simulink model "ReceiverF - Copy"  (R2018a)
settings: Solver=FixedStepDiscrete  StartTime=0.0  StopTime=2  RelTol=1e-3
undefined symbols (not defined in the file): DiscIntNeverNeededParam
libraries: simulink x54, dspsigops x27, commutil2 x6, c280xlib x2, c2803xlib x1, dspstat3 x1

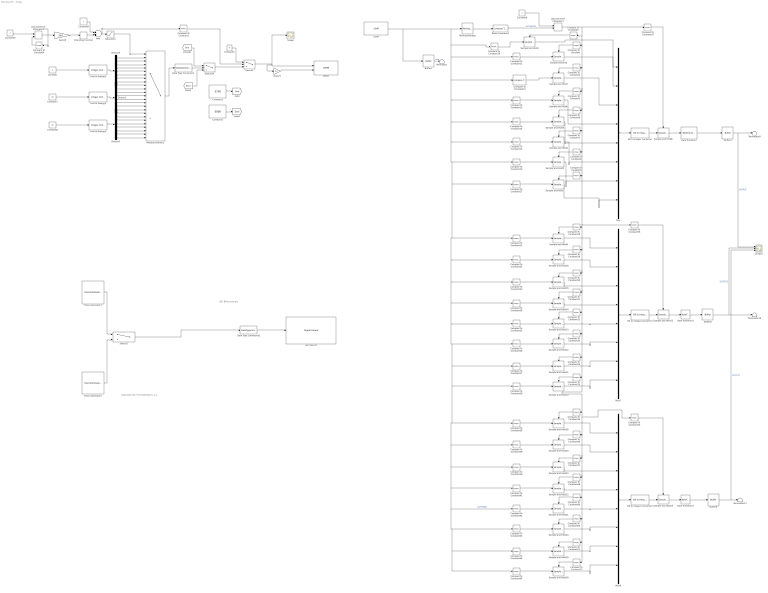
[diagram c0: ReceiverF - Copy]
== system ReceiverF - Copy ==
  note: Copyright 2017 The MathWorks, Inc.
  note: LED Blink example
  Add : Sum
  Bit to Integer Converter : commutil2/Bit to Integer Converter  nbits=8  bitOrder=MSB first  signedOutputValues=Unsigned  outDtype=Inherit via internal rule  outDtypeSigned=Inherit via internal rule
  Bit to Integer Converter4 : commutil2/Bit to Integer Converter  nbits=8  bitOrder=MSB first  signedOutputValues=Unsigned  outDtype=Inherit via internal rule  outDtypeSigned=Inherit via internal rule
  Bit to Integer Converter5 : commutil2/Bit to Integer Converter  nbits=8  bitOrder=MSB first  signedOutputValues=Unsigned  outDtype=Inherit via internal rule  outDtypeSigned=Inherit via internal rule
  Buffer1 : Buffer  N=500  OutputFrames=off
  Buffer4 : Buffer  N=5  OutputFrames=off
  Buffer8 : Buffer  N=5  OutputFrames=off
  Buffer9 : Buffer  N=5  OutputFrames=off
  Compare To Constant : simulink/Logic and Bit Operations/Compare To Constant  relop=>=  const=1  OutDataTypeStr=boolean
  Compare To Constant1 : simulink/Logic and Bit Operations/Compare To Constant  relop=>=  const=25  OutDataTypeStr=boolean
  Compare To Constant10 : simulink/Logic and Bit Operations/Compare To Constant  relop=>=  const=24  OutDataTypeStr=boolean
  Compare To Constant{11..18,21..28,38..45} (24 alike) : simulink/Logic and Bit Operations/Compare To Constant  relop=<=  const=4800  OutDataTypeStr=boolean
  Compare To Constant19 : simulink/Logic and Bit Operations/Compare To Constant  relop=>=  const=8  OutDataTypeStr=boolean
  Compare To Constant2 : simulink/Logic and Bit Operations/Compare To Constant  relop=>=  const=2  OutDataTypeStr=boolean
  Compare To Constant20 : simulink/Logic and Bit Operations/Compare To Constant  relop=>=  const=15  OutDataTypeStr=boolean
  Compare To Constant29 : simulink/Logic and Bit Operations/Compare To Constant  relop=>=  const=9  OutDataTypeStr=boolean
  Compare To Constant3 : simulink/Logic and Bit Operations/Compare To Constant  relop=>=  const=3  OutDataTypeStr=boolean
  Compare To Constant30 : simulink/Logic and Bit Operations/Compare To Constant  relop=>=  const=10  OutDataTypeStr=boolean
  Compare To Constant31 : simulink/Logic and Bit Operations/Compare To Constant  relop=>=  const=11  OutDataTypeStr=boolean
  Compare To Constant32 : simulink/Logic and Bit Operations/Compare To Constant  relop=>=  const=12  OutDataTypeStr=boolean
  Compare To Constant33 : simulink/Logic and Bit Operations/Compare To Constant  relop=>=  const=13  OutDataTypeStr=boolean
  Compare To Constant34 : simulink/Logic and Bit Operations/Compare To Constant  relop=>=  const=14  OutDataTypeStr=boolean
  Compare To Constant35 : simulink/Logic and Bit Operations/Compare To Constant  relop=>=  const=24  OutDataTypeStr=boolean
  Compare To Constant36 : simulink/Logic and Bit Operations/Compare To Constant  relop=>=  const=16  OutDataTypeStr=boolean
  Compare To Constant37 : simulink/Logic and Bit Operations/Compare To Constant  relop=>=  const=23  OutDataTypeStr=boolean
  Compare To Constant4 : simulink/Logic and Bit Operations/Compare To Constant  relop=>  const=1  OutDataTypeStr=uint8
  Compare To Constant46 : simulink/Logic and Bit Operations/Compare To Constant  relop=>=  const=17  OutDataTypeStr=boolean
  Compare To Constant47 : simulink/Logic and Bit Operations/Compare To Constant  relop=>=  const=18  OutDataTypeStr=boolean
  Compare To Constant48 : simulink/Logic and Bit Operations/Compare To Constant  relop=>=  const=19  OutDataTypeStr=boolean
  Compare To Constant49 : simulink/Logic and Bit Operations/Compare To Constant  relop=>=  const=20  OutDataTypeStr=boolean
  Compare To Constant5 : simulink/Logic and Bit Operations/Compare To Constant  relop=>  const=0  OutDataTypeStr=boolean
  Compare To Constant50 : simulink/Logic and Bit Operations/Compare To Constant  relop=>=  const=21  OutDataTypeStr=boolean
  Compare To Constant51 : simulink/Logic and Bit Operations/Compare To Constant  relop=>=  const=22  OutDataTypeStr=boolean
  Compare To Constant52 : simulink/Logic and Bit Operations/Compare To Constant  relop=>=  const=24  OutDataTypeStr=boolean
  Compare To Constant6 : simulink/Logic and Bit Operations/Compare To Constant  relop=>=  const=4  OutDataTypeStr=boolean
  Compare To Constant7 : simulink/Logic and Bit Operations/Compare To Constant  relop=>=  const=5  OutDataTypeStr=boolean
  Compare To Constant8 : simulink/Logic and Bit Operations/Compare To Constant  relop=>=  const=6  OutDataTypeStr=boolean
  Compare To Constant9 : simulink/Logic and Bit Operations/Compare To Constant  relop=>=  const=7  OutDataTypeStr=boolean
  Constant : Constant  Value=6
  Constant1 : Constant  Value=3750  VectorParams1D=off
  Constant2 : Constant  Value=5000  VectorParams1D=off
  Constant4 : Constant
  Constant5 : Constant  Value=0  VectorParams1D=off  SampleTime=-1
  Constant6 : Constant  OutDataTypeStr=int8  SampleTime=-1
  Constant7 : Constant  Value=20  OutDataTypeStr=int8  SampleTime=100e-6
  Constant8 : Constant  Value=33  OutDataTypeStr=int8  SampleTime=100e-6
  Constant9 : Constant  SampleTime=100e-6
  Cost of Energy1 : commutil2/Integer to Bit Converter  nbits=8  signedInputValues=Unsigned  bitOrder=MSB first  outDtype=Inherit via internal rule
  Cost of Energy2 : commutil2/Integer to Bit Converter  nbits=8  signedInputValues=Unsigned  bitOrder=MSB first  outDtype=Inherit via internal rule
  Cost of Energy3 : commutil2/Integer to Bit Converter  nbits=8  signedInputValues=Unsigned  bitOrder=MSB first  outDtype=Inherit via internal rule
  Data Type Conversion : DataTypeConversion  OutDataTypeStr=boolean
  Data Type Conversion1 : DataTypeConversion  Commented=on  OutDataTypeStr=boolean
  Demux1 : Demux  Outputs=8
  Demux2 : Demux  Outputs=8
  Demux3 : Demux  Outputs=8
  Discrete-Time Integrator1 : DiscreteIntegrator  gainval=1e3  ExternalReset=falling  SampleTime=400e-6  ICPrevOutput=DiscIntNeverNeededParam  ICPrevScaledInput=DiscIntNeverNeededParam
  Discrete-Time Integrator2 : DiscreteIntegrator  gainval=1  ExternalReset=rising  SampleTime=100e-6  ShowStatePort=on  ICPrevOutput=DiscIntNeverNeededParam  ICPrevScaledInput=DiscIntNeverNeededParam
  Gain26 : Gain  Gain=1e3
  Gain27 : Gain  Gain=0.5
  LED RIGHT1 : c2803xlib/Digital Output  Commented=on  GPIO_Number=GPIO32~GPIO39  GPIO_Bit0=off  GPIO_BIT0_Toggle=off  GPIO_Bit1=off  GPIO_BIT1_Toggle=off  GPIO_Bit2=on  GPIO_BIT2_Toggle=off  GPIO_Bit3=off  GPIO_BIT3_Toggle=off  GPIO_Bit4=off  GPIO_BIT4_Toggle=off  GPIO_Bit5=off  GPIO_BIT5_Toggle=off  GPIO_Bit6=off  GPIO_BIT6_Toggle=off  GPIO_Bit7=off  GPIO_BIT7_Toggle=off
  Moving Average : dspstat3/Moving Average  Method=Sliding window  ForgettingFactorPort=off  SpecifyWindowLength=on  WindowLength=2  ForgettingFactor=0.9  SimulateUsing=Code generation
  Multiport Switch2 : MultiPortSwitch  Inputs=24
  Mux : Mux  Inputs=8
  Mux7 : Mux  Inputs=8
  Mux8 : Mux  Inputs=8
  Pulse Generator4 : DiscretePulseGenerator  Commented=on  Period=50  PulseWidth=25  SampleTime=0.01
  Pulse Generator5 : DiscretePulseGenerator  Commented=on  Period=50  PulseWidth=25  SampleTime=0.07
  Rate Transition : RateTransition  OutPortSampleTime=1
  Rate Transition1 : RateTransition  OutPortSampleTime=1
  Rate Transition2 : RateTransition  OutPortSampleTime=1
  Reset Condition3 : simulink/Logic and Bit Operations/Compare To Constant  relop=>  const=8e3  OutDataTypeStr=uint8
  Rounding Function : Rounding  Operator=fix
  Sample and Hold{,1..26} (27 alike) : dspsigops/Sample and Hold  trig=Rising edge  initCond=0  latchinput=off
  Saturation : Saturate  UpperLimit=24  LowerLimit=1  RndMeth=Round
  Scope : Scope
  Scope3 : Scope  NumInputPorts=3
  Switch1 : Switch  Criteria=u2 > Threshold
  Switch24 : Switch  Criteria=u2 > Threshold  Threshold=0.5
  Switch3 : Switch  Commented=on  Criteria=u2 > Threshold  Threshold=100
  Terminator{,9..11} (4 alike) : Terminator
  eCAP : c280xlib/eCAP  operatingMode=eCAP  selectCAPx=eCAP1  offsetValue=0  counterSynIn=off  enableCounter=on  syncOutput=CTR=PRD  sampleTime=25e-6  eventPrescaler=0  selectMode=Continuous  enableOneShot=on  stopValue=Capture Event 1  resetEv1Ts=on  ev1Polarity=Rising Edge  resetEv2Ts=off  ev2Polarity=Rising Edge  resetEv3Ts=off  ev3Polarity=Rising Edge  resetEv4Ts=off  ev4Polarity=Rising Edge  tSCntrDataType=single  capEvFlag=off  capFlagDataType=boolean  overFlowFlag=off  overFlowFlagDataType=boolean  periodUnit=Clock cycles  periodSource=Specify via dialog  waveformPeriod=1  dutyUnit=Clock cycles  dutySource=Specify via dialog  dutyCycle=50  outputPolarity=Active High  enableCEVT1Int=off  enableCEVT2Int=off  enableCEVT3Int=off  enableCEVT4Int=off  enableCTROVFInt=off  enablePRDInt=off  enableCMPInt=off
  "ePWM " : c280xlib/ePWM  checkMode=off  useModule=ePWM3  periodUnits=Clock cycles  timerSource=Input port  timerPeriod_clk=3000  timerPeriod_sec=0.0001  tbshadow=Counter equals to zero  countingMode=Up  phaseActiveEnable=Disable  phaseDirection=Count down after sync  phaseActive=0  synchronizationEnable=off  synchronizationOption=Disable  clockPrescale=1  HSclockPrescale=1  ePWMxAStatus=on  CMPAUnits=Clock cycles  CMPASource=Input port  CMPAValue_per=50  CMPAValue_clk=1000  enCMPAshadow=Counter equals to zero  ePWMxAactionLogic1=Set  ePWMxAactionLogic2=Do nothing  ePWMxAactionLogic3=Clear  ePWMxAactionLogic4=Do nothing  ePWMxAactionLogic5=Do nothing  ePWMxAactionLogic6=Do nothing  ePWMxALoadMode=Load on counter equals to zero (CTR=Zero)  ePWMxACSFenable=off  ePWMxACSFvalue=Forcing disable  ePWMxASFreload=Zero  enHRPWM=off  HRPWM_LoadMode=Counter equals to zero (CTR=ZERO)  HRPWM_CTLMode=Phase control mode  HRPWM_EDGMode=Both edge  enSFO=on  ePWMxBStatus=off  CMPBUnits=Clock cycles  CMPBSource=Specify via dialog  CMPBValue_per=50  CMPBValue_clk=32000  enCMPBshadow=Counter equals to zero  ePWMxBactionLogic1=Do nothing  ePWMxBactionLogic2=Set  ePWMxBactionLogic3=Do nothing  ePWMxBactionLogic4=Do nothing  ePWMxBactionLogic5=Clear  ePWMxBactionLogic6=Do nothing  ePWMxBLoadMode=Load on counter equals to zero (CTR=Zero)  ePWMxBCSFenable=off  ePWMxBCSFvalue=Forcing disable  ePWMxBSFreload=Zero  enableDBePWMxA=off  enableDBePWMxB=off  DBpolarity=Active high (AH)  DBedgeDelay=Positive  DBSource_ePWMxA=ePWMxA  DBSource_ePWMxB=ePWMxA  DBperiodSource=Specify via dialog  REDperiod=0  FEDperiod=0  adcstartModuleA=off  adcrequestEventA=First event  adcstartEventA=Counter equals to zero (CTR=Zero)  adcstartModuleB=off  adcrequestEventB=First event  adcstartEventB=Counter equals to zero (CTR=Zero)  intEn=off  intPrd=First event  intSel=Counter equals to zero (CTR=Zero)  chopperEnable=off  chopperFrequency=1  chopperFirstwidth=1  chopperDuty=12.5%  tripZonesource=Specify via dialog  tzselOSHT1=off  tzselOSHT2=off  tzselOSHT3=off  tzselOSHT4=off  tzselOSHT5=off  tzselOSHT6=off  tzselCBC1=off  tzselCBC2=off  tzselCBC3=off  tzselCBC4=off  tzselCBC5=off  tzselCBC6=off  enTzOstIntr=off  enTzCbcIntr=off  ePWMxAforced=No action  ePWMxBforced=No action  timerPeriod=-1  ePWMxAValue=0  ePWMxBValue=0  tripZoneoption=One-shot trip (OSHT)
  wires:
  Reset Condition3/1 -> Discrete-Time Integrator1/2  "ACTIVATOR"
  Moving Average/1 -> Reset Condition3/1
  Constant4/1 -> Discrete-Time Integrator1/1
  Compare To Constant9/1 -> Sample and Hold2/Trigger
  Compare To Constant8/1 -> Sample and Hold3/Trigger
  Compare To Constant7/1 -> Sample and Hold4/Trigger
  Compare To Constant6/1 -> Sample and Hold5/Trigger
  Compare To Constant3/1 -> Sample and Hold6/Trigger
  Compare To Constant2/1 -> Sample and Hold7/Trigger
  Compare To Constant/1 -> Sample and Hold/Trigger
  Sample and Hold2/1 -> Mux/8
  Sample and Hold3/1 -> Mux/7
  Sample and Hold4/1 -> Mux/6
  Sample and Hold5/1 -> Mux/5
  Sample and Hold6/1 -> Mux/4
  Sample and Hold7/1 -> Mux/3
  Sample and Hold/1 -> Mux/2
  Compare To Constant10/1 -> Sample and Hold8/Trigger
  Mux/1 -> Bit to Integer Converter/1
  Bit to Integer Converter/1 -> Sample and Hold8/1
  Sample and Hold8/1 -> Rate Transition/1
  Rate Transition/1 -> Buffer4/1
  Buffer4/1 -> Scope3/1, Terminator9/1  "OUTPUT"
  Compare To Constant11/1 -> Sample and Hold/1
  Compare To Constant12/1 -> Sample and Hold7/1
  Compare To Constant13/1 -> Sample and Hold6/1
  Compare To Constant14/1 -> Sample and Hold5/1
  Compare To Constant15/1 -> Sample and Hold4/1
  Compare To Constant16/1 -> Sample and Hold3/1
  Compare To Constant17/1 -> Sample and Hold2/1
  Compare To Constant25/1 -> Sample and Hold13/1
  Compare To Constant29/1 -> Sample and Hold16/Trigger
  Compare To Constant33/1 -> Sample and Hold12/Trigger
  Compare To Constant20/1 -> Sample and Hold10/Trigger
  Compare To Constant23/1 -> Sample and Hold15/1
  Compare To Constant19/1 -> Sample and Hold9/Trigger
  Compare To Constant34/1 -> Sample and Hold11/Trigger
  Sample and Hold13/1 -> Mux7/5
  Sample and Hold15/1 -> Mux7/3
  Compare To Constant28/1 -> Sample and Hold10/1
  Compare To Constant30/1 -> Sample and Hold15/Trigger
  Sample and Hold12/1 -> Mux7/6
  Compare To Constant27/1 -> Sample and Hold11/1
  Compare To Constant22/1 -> Sample and Hold16/1
  Sample and Hold14/1 -> Mux7/4
  Compare To Constant31/1 -> Sample and Hold14/Trigger
  Sample and Hold10/1 -> Mux7/8
  Mux7/1 -> Bit to Integer Converter4/1
  Compare To Constant32/1 -> Sample and Hold13/Trigger
  Sample and Hold11/1 -> Mux7/7
  Compare To Constant26/1 -> Sample and Hold12/1
  Compare To Constant24/1 -> Sample and Hold14/1
  Sample and Hold16/1 -> Mux7/2
  Compare To Constant21/1 -> Sample and Hold9/1
  Sample and Hold9/1 -> Mux7/1
  Bit to Integer Converter4/1 -> Sample and Hold17/1
  Rate Transition1/1 -> Buffer8/1
  Buffer8/1 -> Scope3/2, Terminator10/1  "OUTPUT2"
  Compare To Constant35/1 -> Sample and Hold17/Trigger
  Sample and Hold26/1 -> Mux8/1
  Compare To Constant38/1 -> Sample and Hold26/1
  Compare To Constant43/1 -> Sample and Hold20/1
  Compare To Constant41/1 -> Sample and Hold22/1
  Compare To Constant52/1 -> Sample and Hold25/Trigger
  Mux8/1 -> Bit to Integer Converter5/1
  Rate Transition2/1 -> Buffer9/1
  Sample and Hold18/1 -> Mux8/8
  Compare To Constant39/1 -> Sample and Hold24/1
  Compare To Constant49/1 -> Sample and Hold21/Trigger
  eCAP/1 -> Buffer1/1, Compare To Constant18/1, Compare To Constant45/1, Compare To Constant44/1, Compare To Constant43/1, Compare To Constant42/1, Compare To Constant41/1, Compare To Constant40/1, Compare To Constant39/1, Compare To Constant38/1, Compare To Constant28/1, Compare To Constant27/1, Compare To Constant26/1, Compare To Constant25/1, Compare To Constant24/1, Compare To Constant23/1, Compare To Constant22/1, Compare To Constant21/1, Compare To Constant17/1, Compare To Constant16/1, Compare To Constant15/1, Compare To Constant14/1, Compare To Constant13/1, Compare To Constant12/1, Compare To Constant11/1, Moving Average/1  "CAPTURED"
  Compare To Constant42/1 -> Sample and Hold21/1
  Sample and Hold22/1 -> Mux8/4
  Compare To Constant44/1 -> Sample and Hold19/1
  Compare To Constant48/1 -> Sample and Hold22/Trigger
  Compare To Constant46/1 -> Sample and Hold24/Trigger
  Sample and Hold25/1 -> Rate Transition2/1
  Sample and Hold20/1 -> Mux8/6
  Compare To Constant47/1 -> Sample and Hold23/Trigger
  Sample and Hold23/1 -> Mux8/3
  Sample and Hold21/1 -> Mux8/5
  Compare To Constant36/1 -> Sample and Hold26/Trigger
  Compare To Constant40/1 -> Sample and Hold23/1
  Compare To Constant45/1 -> Sample and Hold18/1
  Compare To Constant51/1 -> Sample and Hold19/Trigger
  Sample and Hold24/1 -> Mux8/2
  Compare To Constant50/1 -> Sample and Hold20/Trigger
  Sample and Hold19/1 -> Mux8/7
  Compare To Constant37/1 -> Sample and Hold18/Trigger
  Buffer9/1 -> Scope3/3, Terminator11/1  "OUTPUT3"
  Multiport Switch2/1 -> Data Type Conversion/1
  Compare To Constant4/1 -> Discrete-Time Integrator2/2
  Cost of Energy1/1 -> Demux3/1
  Gain26/1 -> Rounding Function/1
  Compare To Constant1/1 -> Switch1/2
  Constant9/1 -> Discrete-Time Integrator2/1
  Constant5/1 -> Switch1/1
  Data Type Conversion/1 -> Switch24/2
  Rounding Function/1 -> Add/2
  Add/1 -> Compare To Constant1/1, Saturation/1
  Switch1/1 -> Scope/1, Gain27/1, "ePWM "/1
  Discrete-Time Integrator2/State -> Compare To Constant4/1
  Cost of Energy2/1 -> Demux1/1
  Cost of Energy3/1 -> Demux2/1
  Discrete-Time Integrator2/1 -> Gain26/1
  Switch24/1 -> Switch1/3
  Saturation/1 -> Multiport Switch2/1
  [One] -> Switch24/1
  Constant2/1 -> [Zero]
  Constant6/1 -> Add/1
  Constant1/1 -> [One]
  Sample and Hold17/1 -> Rate Transition1/1
  Switch3/1 -> Data Type Conversion1/1
  Pulse Generator4/1 -> Switch3/1
  Bit to Integer Converter5/1 -> Sample and Hold25/1
  Data Type Conversion1/1 -> LED RIGHT1/1
  Pulse Generator5/1 -> Switch3/3
  Constant7/1 -> Cost of Energy2/1
  Constant8/1 -> Cost of Energy3/1
  Demux3/1 -> Multiport Switch2/2
  Demux3/2 -> Multiport Switch2/3
  Demux3/3 -> Multiport Switch2/4
  Demux3/4 -> Multiport Switch2/5
  Demux3/5 -> Multiport Switch2/6
  Demux3/6 -> Multiport Switch2/7
  Demux3/7 -> Multiport Switch2/8
  Demux3/8 -> Multiport Switch2/9
  Demux1/1 -> Multiport Switch2/10
  Demux1/2 -> Multiport Switch2/11
  Demux1/3 -> Multiport Switch2/12
  Demux1/4 -> Multiport Switch2/13
  Demux1/5 -> Multiport Switch2/14
  Demux1/6 -> Multiport Switch2/15
  Demux1/7 -> Multiport Switch2/16
  Demux1/8 -> Multiport Switch2/17
  Demux2/1 -> Multiport Switch2/18
  Demux2/2 -> Multiport Switch2/19
  Demux2/3 -> Multiport Switch2/20
  Demux2/4 -> Multiport Switch2/21
  Demux2/5 -> Multiport Switch2/22
  Demux2/6 -> Multiport Switch2/23
  Demux2/7 -> Multiport Switch2/24
  Demux2/8 -> Multiport Switch2/25
  Buffer1/1 -> Terminator/1  "capd"
  Gain27/1 -> "ePWM "/2
  [Zero] -> Switch24/3
  Constant/1 -> Cost of Energy1/1
  Sample and Hold1/1 -> Mux/1
  Compare To Constant5/1 -> Sample and Hold1/Trigger
  Compare To Constant18/1 -> Sample and Hold1/1
  Discrete-Time Integrator1/1 -> Compare To Constant5/1, Compare To Constant52/1, Compare To Constant37/1, Compare To Constant51/1, Compare To Constant50/1, Compare To Constant49/1, Compare To Constant48/1, Compare To Constant47/1, Compare To Constant46/1, Compare To Constant36/1, Compare To Constant20/1, Compare To Constant34/1, Compare To Constant33/1, Compare To Constant32/1, Compare To Constant31/1, Compare To Constant30/1, Compare To Constant29/1, Compare To Constant19/1, Compare To Constant35/1, Compare To Constant9/1, Compare To Constant8/1, Compare To Constant7/1, Compare To Constant6/1, Compare To Constant3/1, Compare To Constant2/1, Compare To Constant/1, Compare To Constant10/1
